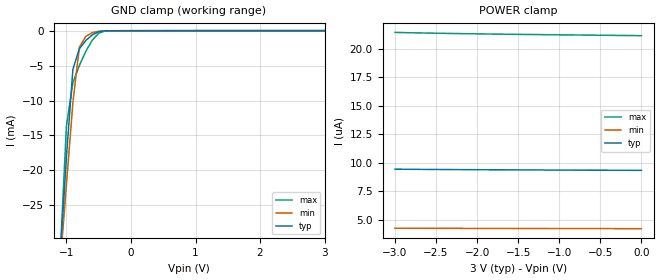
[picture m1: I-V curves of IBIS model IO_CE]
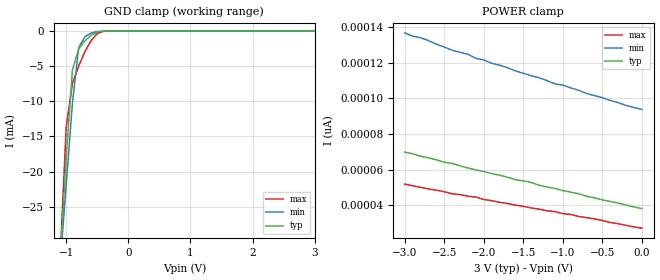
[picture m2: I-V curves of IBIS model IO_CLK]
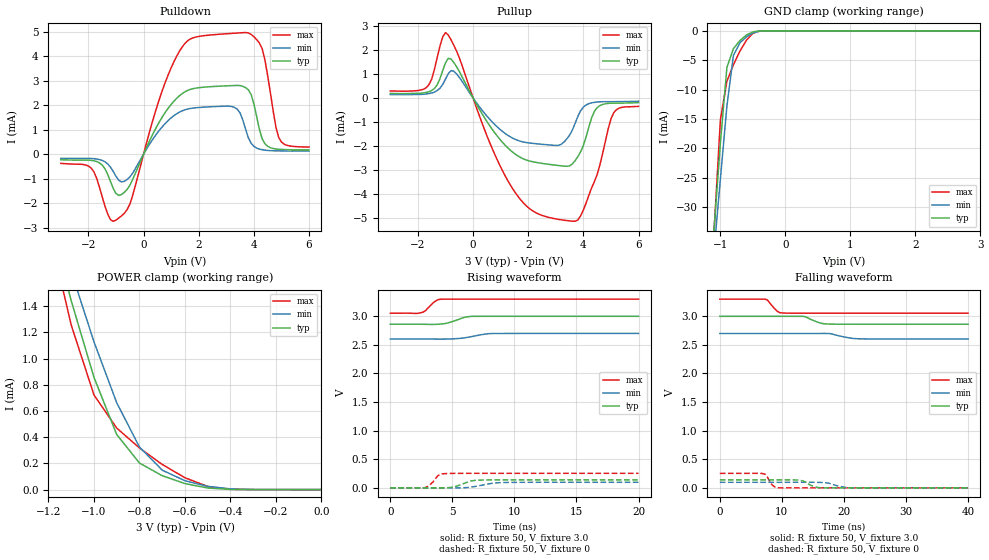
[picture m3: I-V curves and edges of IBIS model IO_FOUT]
[IBIS Ver]   3.2
[Comment Char]   |_char
[File name]   ra4803sa_3.ibs
[File Rev]   1.0
[Date]   Dec 10, 2012
[Source]   This file orginated at SEIKO EPSON Corp.
[Copyright]
   Copyright 2012, SEIKO EPSON Corp.
[Component]   4803sa_3
[Manufacturer]  SEIKO EPSON Corp.
[Package]
| variable   typ   min   max
R_pkg   3.00m   NA   NA
L_pkg   3.70nH   NA   NA
C_pkg   0.70pF   NA   NA
[Pin] signal_name   model_name
1   CE   IO_CE
2   CLK   IO_CLK
3   FOUT   IO_FOUT
4   NC   NC
|5   TEST   IO_TEST
6   VDD   POWER
7   FOE   IO_FOE
8   NC   NC
9   EVIN   IO_STAMP
10   /INT   IO_IRQ
11   VSS   GND
12   T2(VPP)   POWER
13   DO   IO_DIO
14   DI   IO_IN
| Models and submodels in the file (8): IO_CE (Input), IO_CLK (Input), IO_FOUT (3-state), IO_FOE (Input), IO_STAMP (Input), IO_IRQ (Open_drain), IO_DIO (I/O), IO_IN (Input)
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[Model]   IO_CE
Model_type Input
Enable Active-Low
Polarity Non-Inverting
Vinh=2.4
Vinl=0.6
C_comp   5p   4p   6p
[Temperature Range] 25   85   -40
[Voltage Range]   3.0   2.7   3.3
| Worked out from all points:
|   GND clamp passes 1 mA (typ) near -0.65 V on its own axis
[GND Clamp]
-3V       -327.2mA   -271.3mA   -415.9mA
-1.1V     -32.77mA   -33.87mA   -32.85mA
-1V       -18.1mA    -22.01mA   -13.65mA
-900mV    -5.531mA   -10.31mA   -7.443mA
-800mV    -2.587mA   -2.381mA   -4.983mA
-700mV    -1.4mA     -813.2uA   -2.959mA
-600mV    -598.1uA   -285.6uA   -1.36mA
-500mV    -150.1uA   -64.84uA   -354.4uA
-400mV    -19.53uA   -9.583uA   -37.28uA
3V        9.335uA    4.218uA    21.14uA
[POWER Clamp]
-3V       9.439uA    4.255uA    21.45uA
-2.8V     9.427uA    4.25uA     21.42uA
-2.5V     9.412uA    4.244uA    21.38uA
-2.2V     9.399uA    4.239uA    21.34uA
-1.9V     9.388uA    4.235uA    21.31uA
-1.6V     9.378uA    4.231uA    21.29uA
-1.3V     9.37uA     4.228uA    21.26uA
0V        9.335uA    4.215uA    21.16uA
[Model]   IO_CLK
Model_type Input
Enable Active-Low
Polarity Non-Inverting
Vinh=2.4
Vinl=0.6
C_comp   5p   4p   6p
[Temperature Range] 25   85   -40
[Voltage Range]   3.0   2.7   3.3
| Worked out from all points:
|   GND clamp passes 1 mA (typ) near -0.65 V on its own axis
[GND Clamp]
-3V       -321.4mA   -266.3mA   -408.9mA
-1.1V     -32.43mA   -33.46mA   -32.61mA
-1V       -17.96mA   -21.79mA   -13.59mA
-900mV    -5.499mA   -10.22mA   -7.421mA
-800mV    -2.576mA   -2.362mA   -4.965mA
-700mV    -1.392mA   -807.3uA   -2.943mA
-600mV    -591.5uA   -281.9uA   -1.347mA
-500mV    -144.6uA   -61.93uA   -343.6uA
-400mV    -15.25uA   -7.313uA   -28.72uA
3V        38.09pA    97.66pA    24.56pA
[POWER Clamp]
-3V       69.8pA     136.9pA    51.84pA
-2.7V     66.62pA    132.6pA    49.11pA
-2.4V     63.44pA    127.1pA    46.38pA
-2.2V     60.94pA    124.8pA    45.02pA
-2.1V     59.8pA     122.6pA    44.57pA
-2V       58.89pA    121.6pA    43.2pA
-1.4V     52.75pA    112.8pA    38.43pA
-1.3V     51.16pA    111.6pA    37.74pA
-1.1V     49.34pA    108.2pA    36.38pA
-1V       48.2pA     107.5pA    35.24pA
-700mV    45.02pA    102.8pA    32.97pA
0V        38.09pA    93.79pA    27.06pA
[Model]   IO_FOUT
Model_type 3-state
Enable Active-High
Polarity Non-Inverting
Vmeas=1.50
C_comp   5p   4p   6p
[Temperature Range] 25   85   -40
[Voltage Range]   3.0   2.7   3.3
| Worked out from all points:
|   slope of the pulldown table from 0 to 0.45 V, typ, clamps not added: 423 ohm
|   slope of the pullup table from 0 to 0.45 V, typ, clamps not added: 505 ohm
|   GND clamp passes 1 mA (typ) near -0.63 V on its own axis
|   POWER clamp passes 1 mA (typ) near -1.02 V on its own axis
|   falling waveform, R_fixture 50, V_fixture 3.0: 20-80 % time 1.83ns typ, 2.48ns min, 1.19ns max; typ from 3 V to 2.86 V
|   falling waveform, R_fixture 50, V_fixture 0: 20-80 % time 1.47ns typ, 1.96ns min, 883ps max; typ from 0.14 V to 0 V
|   rising waveform, R_fixture 50, V_fixture 3.0: 20-80 % time 1.12ns typ, 1.46ns min, 687ps max; typ from 2.86 V to 3 V
|   rising waveform, R_fixture 50, V_fixture 0: 20-80 % time 1.07ns typ, 1.46ns min, 638ps max; typ from 0 V to 0.14 V
[Pullup]
-3V       187.8uA    140.1uA    293uA
-1.7V     230.8uA    168.1uA    428.9uA
-1V       1.47mA     788.3uA    2.734mA
-700mV    1.485mA    1.12mA     2.209mA
600mV     -1.156mA   -886.4uA   -1.857mA
1.5V      -2.324mA   -1.717mA   -3.907mA
3.1V      -2.826mA   -1.98mA    -5.078mA
3.6V      -2.759mA   -1.341mA   -5.153mA
3.9V      -2.251mA   -535uA     -4.929mA
4.4V      -555.2uA   -183.6uA   -3.497mA
5.1V      -218.2uA   -155.1uA   -618.4uA
6V        -195.2uA   -137.5uA   -351.4uA
[Pulldown]
-3V       -231.2uA   -173.1uA   -379.5uA
-1.9V     -256.8uA   -178.8uA   -570.3uA
-1.2V     -1.12mA    -531.3uA   -2.673mA
-900mV    -1.687mA   -1.067mA   -2.61mA
-500mV    -1.275mA   -934.9uA   -2.045mA
500mV     1.17mA     867.1uA    1.991mA
1.3V      2.38mA     1.711mA    4.194mA
3.1V      2.788mA    1.954mA    4.916mA
3.8V      2.621mA    663.3uA    4.942mA
4.3V      623.7uA    178.1uA    4.299mA
5V        188.2uA    130.1uA    490.7uA
6V        173.2uA    126.6uA    291.1uA
[GND Clamp]
-3V       -337.5mA   -291.8mA   -428.3mA
-1.1V     -34.07mA   -37.78mA   -34.52mA
-1V       -19.07mA   -25.17mA   -15.1mA
-900mV    -6.217mA   -12.77mA   -8.569mA
-800mV    -3.038mA   -4.193mA   -5.779mA
-700mV    -1.663mA   -2.048mA   -3.456mA
-600mV    -716.1uA   -1.013mA   -1.603mA
-500mV    -178.4uA   -369.5uA   -418.8uA
-400mV    -19.08uA   -74.17uA   -35.91uA
3V        64.92pA    794nA      44.45pA
[POWER Clamp]
-3V       16.1mA     14.22mA    19.24mA
-1.2V     2.101mA    2.242mA    2.001mA
-1.1V     1.442mA    1.665mA    1.256mA
-1V       856.8uA    1.128mA    722.6uA
-900mV    420.7uA    663uA      469.5uA
-800mV    202.7uA    324.8uA    317.8uA
-700mV    106.2uA    148.3uA    192.1uA
-600mV    46.01uA    67.7uA     90.33uA
-500mV    12.08uA    24.6uA     23.88uA
-400mV    1.58uA     5.546uA    2.09uA
0V        64.92pA    1.18nA     51.84pA
[Falling Waveform]
R_fixture=50
V_fixture=3.0
V_fixture_min=2.7
V_fixture_max=3.3
0s        3V         2.7V       3.3V
7.273ns   3V         2.7V       3.3V
7.677ns   3V         2.7V       3.284V
9.293ns   3V         2.7V       3.085V
10.1ns    3V         2.7V       3.058V
13.74ns   2.994V     2.7V       3.054V
16.16ns   2.883V     2.7V       3.054V
17.37ns   2.866V     2.7V       3.054V
22.22ns   2.861V     2.608V     3.054V
40ns      2.861V     2.603V     3.054V
[Falling Waveform]
R_fixture=50
V_fixture=0
V_fixture_min=0
V_fixture_max=0
0s        139.6mV    97.41mV    253.4mV
7.273ns   139.7mV    97.4mV     240.3mV
8.081ns   139.7mV    97.41mV    96.44mV
8.485ns   139.8mV    97.41mV    46.72mV
9.293ns   139.9mV    97.43mV    1.252mV
12.93ns   132mV      97.74mV    2.138uV
14.95ns   32.01mV    97.93mV    1.944uV
16.57ns   470.2uV    93.46mV    2.243uV
21.01ns   -9.897uV   2.098mV    1.936uV
40ns      10.23uV    -4.216uV   2.36uV
[Rising Waveform]
R_fixture=50
V_fixture=3.0
V_fixture_min=2.7
V_fixture_max=3.3
0s        2.861V     2.603V     3.054V
2.424ns   2.861V     2.603V     3.06V
2.828ns   2.859V     2.603V     3.096V
3.636ns   2.858V     2.601V     3.265V
4.04ns    2.864V     2.6V       3.298V
4.646ns   2.885V     2.602V     3.3V
5.455ns   2.942V     2.611V     3.3V
6.465ns   2.998V     2.642V     3.3V
8.283ns   3V         2.699V     3.3V
20ns      3V         2.7V       3.3V
[Rising Waveform]
R_fixture=50
V_fixture=0
V_fixture_min=0
V_fixture_max=0
0s        0V         0V         0V
2.828ns   73.78uV    16.66uV    5.172mV
3.434ns   -1.982uV   56.73uV    102.2mV
3.838ns   -165.2uV   41.61uV    213.3mV
4.242ns   -545.4uV   -6.788uV   246mV
5.051ns   13.72mV    -258.8uV   252.7mV
6.465ns   118.5mV    11.93mV    253.4mV
7.071ns   134.2mV    33.36mV    253.3mV
9.495ns   139.5mV    94.3mV     253.4mV
20ns      139.6mV    97.41mV    253.4mV
[Ramp]
R_load=50
dV/dt_r   8.379E-2/1.051E-9   5.845E-2/1.453E-9   1.520E-1/6.195E-10
dV/dt_f   8.310E-2/1.820E-9   3.599E-2/1.290E-9   1.474E-1/1.156E-9
|[End   IO_FOUT
